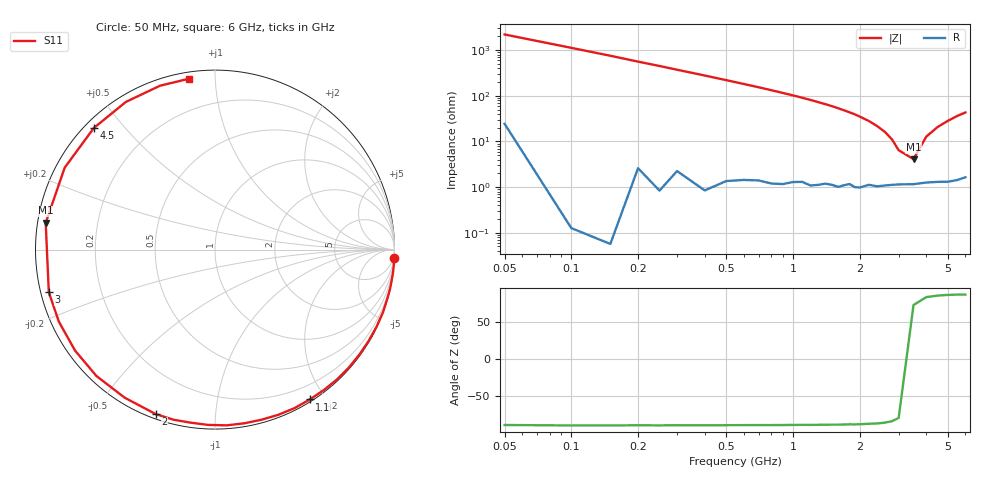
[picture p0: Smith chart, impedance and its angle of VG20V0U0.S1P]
! Infineon Technologies  Discrete & RF Semiconductors
! BB 831
! Si Tuning Diode in SOD323
! VR = 20 V
! S-Parameters:  July  1999
# GHz  S  MA  R  50
!  f  S11
! GHz  MAG  ANG
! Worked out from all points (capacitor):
!   34 points, 50 MHz to 6 GHz, reference 50 ohm
!   read as one part to ground: C = 1.42 pF near 50 MHz
!   lowest |Z| = 4.1 ohm at 3.5 GHz (marker M1)
!   series resonance near 3.308 GHz, so ESL is about 1.6 nH
!   S11 on the Smith chart (normalised r, x): 50 MHz: 0, -44; 1.1 GHz: 0.03, -1.81; 2 GHz: 0.02, -0.70; 3 GHz: 0.02, -0.13; 4.5 GHz: 0.03, +0.41; 6 GHz: 0.03, +0.86
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0.05  0.9995 -2.6
0.15  1 -7.6
0.25  0.9996 -12.7
0.4  0.9989 -20.4
0.6  0.996 -30.8
0.7  0.9947 -36.0
0.8  0.994 -41.4
0.9  0.9927 -46.8
1.1  0.9879 -57.7
1.2  0.9881 -63.3
1.3  0.9858 -69.0
1.5  0.9815 -80.3
1.6  0.9813 -86.2
1.7  0.9774 -92.2
1.8  0.9737 -98.0
1.9  0.9756 -103.7
2  0.9741 -109.8
2.2  0.9664 -121.4
2.4  0.9656 -133.2
2.6  0.9615 -144.2
2.8  0.9581 -155.2
3  0.9559 -165.6
3.5  0.955 171.0
4  0.9538 151.4
4.5  0.9565 134.9
5  0.961 121.1
5.5  0.9631 108.5
6  0.9631 98.5
